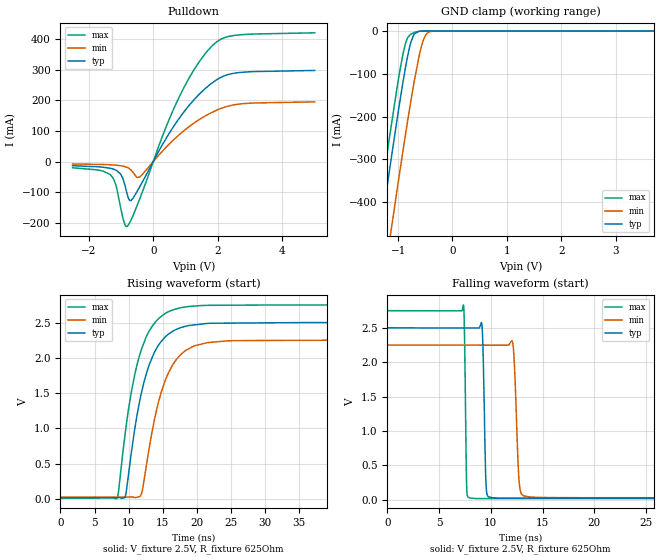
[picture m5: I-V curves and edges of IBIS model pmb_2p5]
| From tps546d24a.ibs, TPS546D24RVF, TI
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|   pmb_2p5 Model
[Model]   pmb_2p5
Model_type   I/O_open_drain
Polarity   Inverting
Enable   Active-High
Vinl = 0.8
Vinh = 1.35
Vmeas = 1.25
Vref = 2.5
Cref = 2pF
Rref = 625
|   typ   min   max
C_comp   3.370pF   3.309pF   3.433pF
|C_comp_pull_down   3.959pF   3.799pF   4.402pF
|  Where Nom  PVT is Nominal Process, 2.5V,   25C
|   Fast PVT is Strong Process,  2.75V, -40C
|   Slow PVT is Weak Process,   2.25V, 150C
[Voltage Range]   2.5   2.25   2.75
|Junction Temperature
[Temperature Range]   25   150   -40
[Pullup Reference]   2.5   2.25   2.75
[Pulldown Reference]   0   0   0
[Power Clamp Reference]   2.5   2.25   2.75
[GND Clamp Reference]   0   0   0
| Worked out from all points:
|   slope of the pulldown table from 0 to 0.375 V, typ, clamps not added: 5.24 ohm
|   GND clamp passes 1 mA (typ) near -0.62 V on its own axis
|   falling waveform, V_fixture 2.5V, R_fixture 625Ohm: 20-80 % time 200ps typ, 324ps min, 139ps max; typ from 2.5 V to 0.019 V
|   rising waveform, V_fixture 2.5V, R_fixture 625Ohm: 20-80 % time 3.25ns typ, 3.34ns min, 3.17ns max; typ from 0.019 V to 2.5 V
[Pulldown]
|   Voltage   I(typ)   I(min)   I(max)
-2.5V     -13.72mA   -8.053mA   -20.46mA
-1.323V   -22.39mA   -10.74mA   -43.88mA
-1.165V   -27.82mA   -11.86mA   -74.18mA
-1.015V   -40.8mA    -13.66mA   -148.8mA
-820mV    -102mA     -18.78mA   -213.1mA
-692.5mV  -128.4mA   -27.25mA   -192.4mA
-422.5mV  -83.21mA   -51.04mA   -123.2mA
747.5mV   133.1mA    82.56mA    198.9mA
1.28V     204.4mA    127.3mA    303.7mA
1.798V    255.5mA    159.9mA    376.1mA
2.533V    289.7mA    186.3mA    413.3mA
5V        298.3mA    195.5mA    421.6mA
[GND Clamp]
|   Voltage   I(typ)   I(min)   I(max)
-2.5V     -1.553A    -1.708A    -1.484A
-1.51V    -638.6mA   -803.9mA   -562.4mA
-1.225V   -383.6mA   -550.1mA   -306.3mA
-1.157V   -324.5mA   -491mA     -247.5mA
-1.015V   -203.1mA   -367.8mA   -128.8mA
-910mV    -119mA     -279.4mA   -53.29mA
-827.5mV  -60.26mA   -212.1mA   -16.51mA
-707.5mV  -7.259mA   -120.3mA   -3.586mA
-542.5mV  -94.15uA   -23.9mA    -109.9uA
-475mV    -15.2uA    -6.464mA   -14.9uA
-385mV    -975.9nA   -666uA     -535.6nA
5V        0A         0A         0A
[POWER Clamp]
|   Voltage   I(typ)   I(min)   I(max)
-2.5V     0A         0A         0A
0V        0A         0A         0A
5V        0A         0A         0A
[Ramp]
R_load = 625
|   typ   min   max
dV/dt_r   1.48831/3.22947e-09   1.33301/3.33167e-09   1.64144/3.15247e-09
dV/dt_f   1.48831/1.99842e-10   1.33301/3.24027e-10   1.64144/1.39421e-10
[Falling Waveform]
V_fixture = 2.5V
V_fixture_min = 2.25V
V_fixture_max = 2.75V
R_fixture = 625Ohm
C_fixture = 0F
|   Time   V(typ)   V(min)   V(max)
0s        2.5V       2.25V      2.75V
7.357ns   2.498V     2.249V     2.834V
7.69ns    2.498V     2.248V     121.6mV
8.597ns   2.497V     2.248V     16.12mV
9.154ns   2.525V     2.248V     16.12mV
9.608ns   95.92mV    2.248V     16.12mV
10.78ns   22mV       2.248V     16.11mV
12.86ns   21.99mV    124.3mV    16.11mV
14.68ns   21.98mV    31.76mV    16.1mV
500ns     19.48mV    28.31mV    14.27mV
[Rising Waveform]
V_fixture = 2.5V
V_fixture_min = 2.25V
V_fixture_max = 2.75V
R_fixture = 625Ohm
C_fixture = 0F
|   Time   V(typ)   V(min)   V(max)
0s        19.48mV    28.31mV    14.27mV
8.353ns   20.16mV    28.31mV    12.86mV
9.561ns   50.72mV    28.31mV    969.9mV
10.49ns   718mV      28.82mV    1.563V
11.71ns   1.425V     39.78mV    2.066V
13.03ns   1.901V     719.7mV    2.38V
15.44ns   2.302V     1.695V     2.632V
17.82ns   2.433V     2.061V     2.713V
20.54ns   2.476V     2.191V     2.74V
500ns     2.5V       2.25V      2.75V
